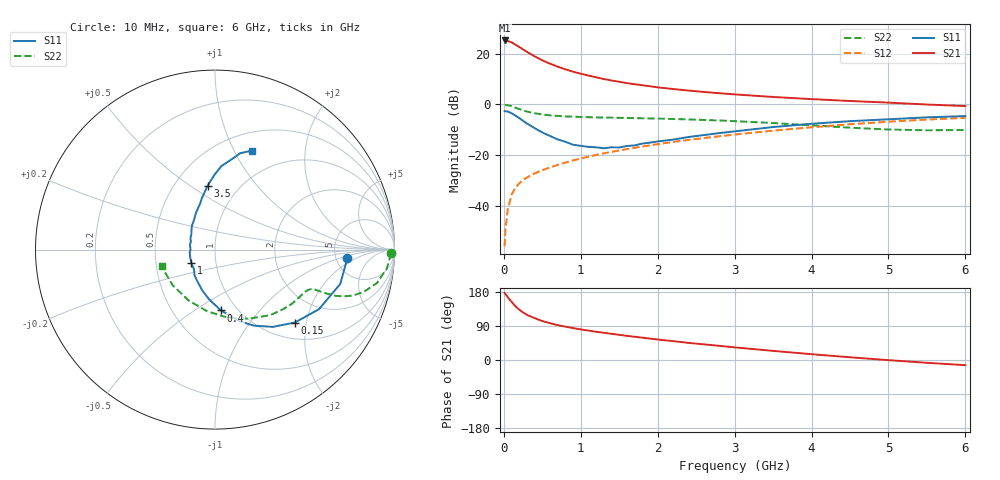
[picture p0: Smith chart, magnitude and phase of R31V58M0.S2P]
! SIEMENS Small Signal Semiconductors
! BFR181
! Si NPN RF Bipolar Junction Transistor in SOT23
! VCE = 1.5 V  IC = 8 mA
! Common Emitter S-Parameters:  May  1996
# GHz  S  MA  R  50
!  f  S11  S21  S12  S22
! GHz  MAG  ANG  MAG  ANG  MAG  ANG  MAG  ANG
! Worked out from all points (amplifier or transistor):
!   36 points, 10 MHz to 6 GHz, reference 50 ohm
!   highest |S21| = 25.2 dB at 10 MHz (marker M1)
!   |S21| within 3 dB of that: start of sweep to 222.9 MHz
!   unconditionally stable (mu >= 1): 718.7 MHz to 2.847 GHz
!   at 250 MHz: K = 0.58, MSG = 25.7 dB, |S12| = -29.8 dB
!   at 1.4 GHz: K = 1.10, MAG = 12.2 dB, |S12| = -18.7 dB
!   at 6 GHz: K = 0.87, MSG = 2.3 dB, |S12| = -5.3 dB
!   S11 on the Smith chart (normalised r, x): 10 MHz: 6.37, -1.30; 150 MHz: 1.35, -1.72; 400 MHz: 0.84, -0.65; 1 GHz: 0.76, -0.12; 3.5 GHz: 0.72, +0.59; 6 GHz: 0.70, +1.18
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0.01  0.7381 -3.6  18.22 177.1  0.0016 91.3  0.9785 -1.2
0.02  0.733 -6.4  18.04 174.1  0.0033 84.4  0.9754 -2.6
0.05  0.7237 -15.3  17.79 166.2  0.0083 83.3  0.9632 -6.3
0.1  0.6679 -29.8  16.69 153.6  0.0165 75.7  0.9207 -11.7
0.15  0.6024 -42.4  15.1 141.8  0.0228 70.9  0.8613 -15.9
0.2  0.5378 -53.2  13.59 133.1  0.0278 68.1  0.8103 -18.4
0.25  0.4741 -63.2  12.13 125.3  0.0323 65.9  0.7627 -20.0
0.3  0.42 -71.3  10.85 119.2  0.0362 65.1  0.7226 -20.9
0.4  0.3407 -84.4  8.871 110.5  0.0436 64.9  0.6695 -21.5
0.5  0.2792 -96.7  7.381 102.8  0.0503 65.1  0.633 -21.7
0.6  0.2386 -107.2  6.339 97.1  0.057 65.9  0.6083 -21.7
0.7  0.204 -118.3  5.552 92.1  0.0641 66.8  0.5925 -22.0
0.8  0.1828 -128.5  4.911 88.0  0.071 66.8  0.5805 -22.3
1  0.1521 -150.3  4.026 80.7  0.0854 67.6  0.5654 -23.5
1.1  0.1453 -161.0  3.7 77.7  0.0931 67.9  0.5589 -24.3
1.3  0.1363 179.0  3.161 71.8  0.1084 67.9  0.5502 -26.1
1.6  0.1514 154.5  2.632 63.7  0.1314 67.4  0.5398 -29.4
2.2  0.202 125.3  2.007 49.8  0.1815 64.7  0.5153 -37.8
3.5  0.3574 96.7  1.4 24.1  0.3028 54.3  0.4283 -64.1
4.5  0.4667 85.6  1.167 7.2  0.4054 42.9  0.347 -97.0
5.5  0.5553 75.3  0.994 -7.4  0.5027 29.3  0.3083 -140.0
6  0.5877 69.7  0.925 -13.6  0.5443 21.9  0.3125 -162.5
